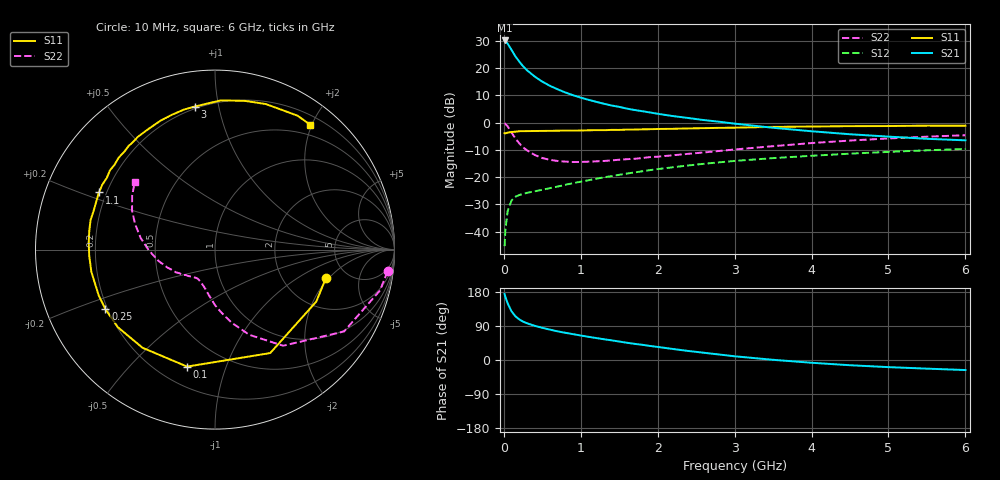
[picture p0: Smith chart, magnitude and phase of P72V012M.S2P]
! SIEMENS Small Signal Semiconductors
! BFP196
! Si NPN RF Bipolar Junction Transistor in SOT143
! VCE = 2 V  IC = 12 mA
! Common Emitter S-Parameters:  May  1996
# GHz  S  MA  R  50
!  f  S11  S21  S12  S22
! GHz  MAG  ANG  MAG  ANG  MAG  ANG  MAG  ANG
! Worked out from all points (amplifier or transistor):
!   36 points, 10 MHz to 6 GHz, reference 50 ohm
!   highest |S21| = 30.1 dB at 10 MHz (marker M1)
!   |S21| within 3 dB of that: start of sweep to 89.78 MHz
!   unconditionally stable (mu >= 1): 814.2 MHz to 3.406 GHz
!   at 250 MHz: K = 0.46, MSG = 23.4 dB, |S12| = -26.2 dB
!   at 1.4 GHz: K = 1.14, MAG = 10.7 dB, |S12| = -19.7 dB
!   at 6 GHz: K = 0.98, MSG = 1.6 dB, |S12| = -9.7 dB
!   S11 on the Smith chart (normalised r, x): 10 MHz: 3.47, -1.86; 100 MHz: 0.31, -0.74; 250 MHz: 0.19, -0.25; 1.1 GHz: 0.17, +0.23; 3 GHz: 0.19, +0.85; 6 GHz: 0.33, +1.97
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0.01  0.6381 -14.4  32.04 174.0  0.0054 85.1  0.9693 -7.2
0.02  0.6343 -27.2  30.89 166.5  0.0108 78.0  0.9471 -13.9
0.05  0.6534 -61.9  27.93 149.2  0.0239 63.1  0.8515 -32.4
0.1  0.6701 -103.4  21.5 128.4  0.0373 47.7  0.6562 -54.7
0.15  0.6798 -126.4  16.38 115.5  0.0435 39.9  0.5114 -68.1
0.2  0.6927 -141.3  13.15 107.2  0.0469 36.4  0.4166 -77.3
0.25  0.695 -151.4  10.76 101.3  0.049 34.4  0.3503 -84.5
0.3  0.6964 -158.5  9.13 97.0  0.0513 34.5  0.3098 -89.9
0.4  0.6999 -169.8  7 90.3  0.0548 35.3  0.2546 -97.9
0.5  0.7016 -177.1  5.624 85.0  0.0584 37.1  0.223 -104.4
0.6  0.7047 176.8  4.714 80.1  0.0627 39.2  0.2067 -109.7
0.7  0.7083 171.4  4.064 75.6  0.067 40.6  0.197 -113.8
0.8  0.7125 166.7  3.559 71.8  0.0723 41.9  0.1921 -117.6
1.1  0.7209 153.8  2.614 61.2  0.0874 44.9  0.1916 -125.6
1.3  0.7234 146.3  2.215 54.8  0.0989 45.7  0.1974 -130.7
1.6  0.742 136.3  1.801 45.5  0.1159 45.7  0.2126 -137.2
2.2  0.768 118.6  1.313 29.0  0.1514 42.4  0.2513 -149.6
3  0.8051 98.0  0.955 9.8  0.1976 34.6  0.3202 -168.4
3.5  0.8323 87.7  0.802 0.5  0.2226 29.0  0.3687 -179.3
4.5  0.8588 70.8  0.61 -13.8  0.2687 18.0  0.4672 162.3
5.5  0.8765 58.3  0.503 -22.8  0.3096 6.8  0.5506 147.0
6  0.8749 52.8  0.472 -26.5  0.3279 0.7  0.5854 139.8
